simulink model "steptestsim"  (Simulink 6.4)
settings: Solver=ode23s  StartTime=0.0  StopTime=400  MaxStep=0.05  RelTol=1e-8
libraries: simulink x1, cstblocks x1

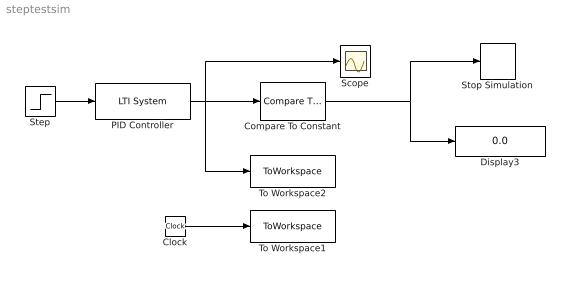
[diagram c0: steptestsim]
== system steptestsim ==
  Clock : Clock
  Compare To Constant : simulink/Logic and Bit Operations/Compare To Constant  SystemSampleTime=-1  relop=>=  const=1-exp(-1)  LogicOutDataTypeMode=boolean  ZeroCross=off
  Display3 : Display
  PID Controller : cstblocks/LTI System  SystemSampleTime=-1  sys=syst  IC=[]
  Scope : Scope
  Step : Step  Time=0  SampleTime=0
  Stop Simulation : Stop
  To Workspace1 : ToWorkspace  VariableName=tid  SampleTime=-1  SaveFormat=Array
  To Workspace2 : ToWorkspace  VariableName=step_vals  SampleTime=-1  SaveFormat=Array
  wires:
  Clock/1 -> To Workspace1/1
  Step/1 -> PID Controller/1
  PID Controller/1 -> To Workspace2/1, Compare To Constant/1, Scope/1
  Compare To Constant/1 -> Stop Simulation/1, Display3/1
